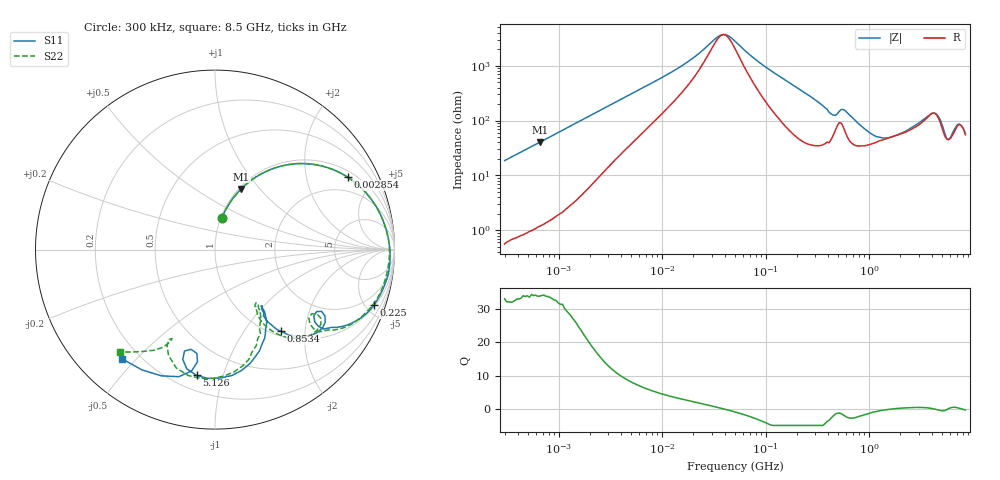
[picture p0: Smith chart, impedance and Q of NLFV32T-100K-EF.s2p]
! S-parameter Generated by TDK Corporation
! Copyright(C) 2015 TDK Corporation.
! All Rights Reserved.
! TDK P/N: NLFV32T-100K-EF (Inductors)
! Property: L=10uH at 2.52MHz
! Size(LxWxT): 3.2x2.5x2.2mm, 0.126x0.098x0.087inches
! Model Type: s2p (Touchstone File Format Version 1.0)
! Frequency: DC=Yes Start=0.3MHz Stop=8500MHz 225points Log-sweep
! Note:
! Model Generated on Jun. 23, 2015
! Hash(MD5):
! Port Assignments:
!  1 ---@@@--- 2
! Applicable Conditions:
!  Temperature = 25 degC
!  DC Bias Current = 0 A
!  Small Signal Operation
! Terms and conditions regarding TDK Simulation Models
! (1)This simulation model is being provided solely for informational purposes. Please refer to the specifications of the products in terms of detailed characteristics of such products.
! (2)In no event shall TDK Corporation of any of its subsidiaries be liable for any loss or damage arising, directly or indirectly,
!  From any information contained in this simulation model, including, but not limited to loss or damages arising from any inaccuracies, omissions or errors in connection with such information.
! (3)Any and all copyrights on this simulation model are owned by TDK Corporation.
!  Duplication or redistribution of this simulation model without prior written permission from TDK Corporation is prohibited.
! (4)This simulation model is subject to any modification or change without any prior notice.
! (5)Neither TDK Corporation nor any of its subsidiaries shall make any warranty, express or implied,
!  Including but not limited to the correctness, implied warranties of merchantability and fitness for a particular purpose with respect to this simulation models.
! (6)The use of this simulation model shall be deemed to have consented to the terms and conditions hereof.
# MHz S MA R 50
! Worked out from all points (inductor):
!   224 points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, 300 kHz to 8.5 GHz, reference 50 ohm
!   read as one part in series: L = 9.83 uH near 314.1 kHz
!   highest Q = 34.1 at 655.4 kHz (marker M1), where L = 9.76 uH
!   self-resonance near 38.94 MHz
!   S11 on the Smith chart (normalised r, x): 300 kHz: 1.01, +0.37; 2.854 MHz: 1.26, +3.49; 225 MHz: 1.11, -5.67; 853.4 MHz: 1.08, -1.49; 5.126 GHz: 0.29, -0.82; 8.5 GHz: 0.14, -0.46
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0.3  0.1807 77.9  0.9758 -10.4  0.9807 -10.7  0.1796 77.9
0.6554417  0.3683 66.7  0.9192 -21.6  0.9208 -22.0  0.3679 66.7
1.72111  0.7101 42.2  0.6742 -45.2  0.6754 -45.5  0.7107 42.2
2.853835  0.8417 28.7  0.4832 -57.1  0.4839 -57.5  0.8423 28.6
9.430415  0.9527 9.1  0.1652 -68.9  0.1653 -69.2  0.9528 8.9
35.77084  0.9745 -0.2  0.02763 -16.4  0.02765 -16.7  0.9722 -0.5
41.06062  0.9753 -1.0  0.02645 9.2  0.02648 8.9  0.9725 -1.3
51.67171  0.9765 -2.4  0.03614 43.0  0.03616 42.7  0.972 -2.8
93.92989  0.976 -6.9  0.09419 68.2  0.09424 67.8  0.9667 -7.5
224.9819  0.9371 -19.3  0.2648 63.3  0.2649 62.9  0.9258 -20.4
283.1228  0.9015 -24.6  0.3382 57.0  0.3383 56.7  0.8883 -25.9
448.3627  0.6867 -35.9  0.5068 29.4  0.5073 28.9  0.6728 -38.1
564.2308  0.7355 -33.4  0.4291 29.2  0.429 28.9  0.7224 -35.3
853.3868  0.5834 -51.2  0.6201 15.2  0.6214 14.8  0.5693 -54.4
1551.304  0.4112 -50.7  0.6342 -17.1  0.6345 -17.9  0.3801 -53.9
2456.696  0.4487 -51.8  0.5492 -41.3  0.5488 -42.0  0.4241 -54.1
3548.748  0.5885 -63.6  0.3943 -59.8  0.3953 -60.3  0.5824 -66.7
4465.833  0.7082 -82.4  0.2998 -52.0  0.2997 -52.5  0.7055 -85.8
5126.239  0.7082 -98.3  0.3588 -45.1  0.3583 -45.5  0.7174 -102.1
6161.135  0.5715 -103.5  0.4448 -72.7  0.4401 -72.9  0.5602 -116.9
7072.242  0.6892 -101.0  0.3039 -89.0  0.3051 -89.8  0.6149 -117.9
8500  0.799 -130.4  0.2349 -79.1  0.2344 -78.3  0.7767 -132.7
